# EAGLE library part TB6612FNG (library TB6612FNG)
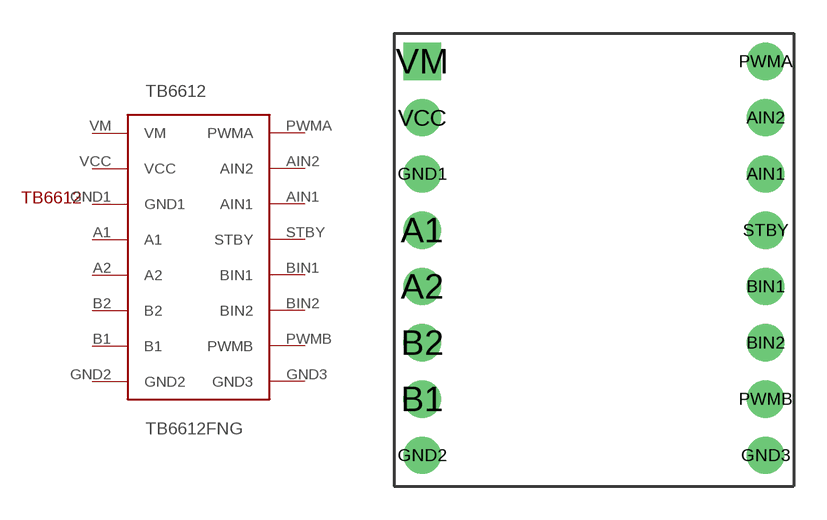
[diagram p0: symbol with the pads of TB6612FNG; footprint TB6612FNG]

Designator prefix TB6612

## TB6612FNG  [TB6612FNG]
A1  A1
A2  A2
AIN1  AIN1
AIN2  AIN2
B1  B1
B2  B2
BIN1  BIN1
BIN2  BIN2
GND1  GND1
GND2  GND2
GND3  GND3
PWMA  PWMA
PWMB  PWMB
STBY  STBY
VCC  VCC
VM  VM

## Footprint TB6612FNG (pad centres in mm)
drill 0.6 pad 1.676: A1 -7.62,-1.27; A2 -7.62,-3.81; AIN1 7.874,1.27; AIN2 7.874,3.81; B1 -7.62,-8.89; B2 -7.62,-6.35; BIN1 7.874,-3.81; BIN2 7.874,-6.35; GND1 -7.62,1.27; GND2 -7.62,-11.43; GND3 7.874,-11.43; PWMA 7.874,6.35; PWMB 7.874,-8.89; STBY 7.874,-1.27; VCC -7.62,3.81
drill 0.7 pad 1.676 square: VM -7.62,6.35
